FUNCTION_BLOCK FB_DO_IED_LD1_LEDGGIO7_AnOut1 EXTENDS FB_AcsiCommonControllableDataClass
VAR_INPUT
	mxVal: FB_AcsiDATypeAnalogueValue := (fc:=ACSI_FC_MX, TrgOp:=ACSI_TrgOp_dchg, bLinkResult:=THIS^.AddDataToContainer(ipData:=mxVal));
	q: FB_AcsiDATypeQuality := (fc:=ACSI_FC_MX, TrgOp:=ACSI_TrgOp_qchg, bLinkResult:=THIS^.AddDataToContainer(ipData:=q));
	t: FB_AcsiDATypeTimeStamp := (fc:=ACSI_FC_MX, bLinkResult:=THIS^.AddDataToContainer(ipData:=t));
	stSeld: FB_AcsiBATypeBOOLEAN := (fc:=ACSI_FC_MX, TrgOp:=ACSI_TrgOp_dchg, bLinkResult:=THIS^.AddDataToContainer(ipData:=stSeld));
	ctlModel: FB_AcsiDATypeCtlModels := (fc:=ACSI_FC_CF, TrgOp:=ACSI_TrgOp_dchg, eValue:=E_AcsiCtlModels.SBOWithEnhancedSecurity, bLinkResult:=THIS^.AddDataToContainer(ipData:=ctlModel));
	sboTimeout: FB_AcsiBATypeINT32U := (fc:=ACSI_FC_CF, TrgOp:=ACSI_TrgOp_dchg, nValue:=30000, bLinkResult:=THIS^.AddDataToContainer(ipData:=sboTimeout));
	sboClass: FB_AcsiDATypeSboClasses := (fc:=ACSI_FC_CF, TrgOp:=ACSI_TrgOp_dchg, eValue:=E_AcsiSboClasses.OperateOnce, bLinkResult:=THIS^.AddDataToContainer(ipData:=sboClass));
	units: FB_AcsiDATypeUnit := (fc:=ACSI_FC_CF, TrgOp:=ACSI_TrgOp_dchg, SIUnit:=(eValue:=E_AcsiSIUnit.Volt), multiplier:=(eValue:=E_AcsiMultiplier.Milli, bPresence:=TRUE), bLinkResult:=THIS^.AddDataToContainer(ipData:=units));
	operTimeout: FB_AcsiBATypeINT32U := (fc:=ACSI_FC_CF, TrgOp:=ACSI_TrgOp_dchg, nValue:=30000, bLinkResult:=THIS^.AddDataToContainer(ipData:=operTimeout));
	Oper: FB_AcsiCDC_Oper_AnalogueValue := (fc:=ACSI_FC_CO, bLinkResult:=THIS^.AddDataToContainer(ipData:=Oper));
	SBOw: FB_AcsiCDC_SBOw_AnalogueValue := (fc:=ACSI_FC_CO, bLinkResult:=THIS^.AddDataToContainer(ipData:=SBOw));
	Cancel: FB_AcsiCDC_Cancel_AnalogueValue := (fc:=ACSI_FC_CO, bLinkResult:=THIS^.AddDataToContainer(ipData:=Cancel));
	
	fbControl: FB_SboControl := (ipCtrl:=THIS^.AddServerJob(ipEvent:=fbControl, ipCompletion:=fbControl), eType:=E_AcsiCDCType.APC, ipBehVal:=fbIED.IEDLD1.LEDGGIO7.Beh.stVal);
END_VAR
VAR
END_VAR

END_FUNCTION_BLOCK
